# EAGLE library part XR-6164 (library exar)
CCITT G.703 CO-DIRECTIONAL INTERFACE
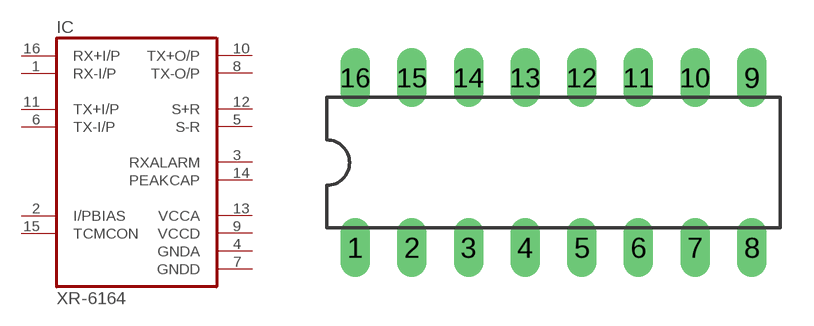
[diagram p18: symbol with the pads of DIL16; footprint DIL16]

Designator prefix IC

## XR-6164 (OC_FARNELL: unknown; OC_NEWARK: unknown)  [DIL16]
1  RX-I/P  in
2  I/PBIAS  in
3  RXALARM  out
4  GNDA  pwr
5  S-R  out
6  TX-I/P  in
7  GNDD  pwr
8  TX-O/P  out
9  VCCD  pwr
10  TX+O/P  out
11  TX+I/P  in
12  S+R  out
13  VCCA  pwr
14  PEAKCAP  out
15  TCMCON  in
16  RX+I/P  in

## Footprint DIL16 (pad centres in mm)
Dual In Line Package
drill 0.813 long: 1 -8.89,-3.81; 2 -6.35,-3.81; 3 -3.81,-3.81; 4 -1.27,-3.81; 5 1.27,-3.81; 6 3.81,-3.81; 7 6.35,-3.81; 8 8.89,-3.81; 9 8.89,3.81; 10 6.35,3.81; 11 3.81,3.81; 12 1.27,3.81; 13 -1.27,3.81; 14 -3.81,3.81; 15 -6.35,3.81; 16 -8.89,3.81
